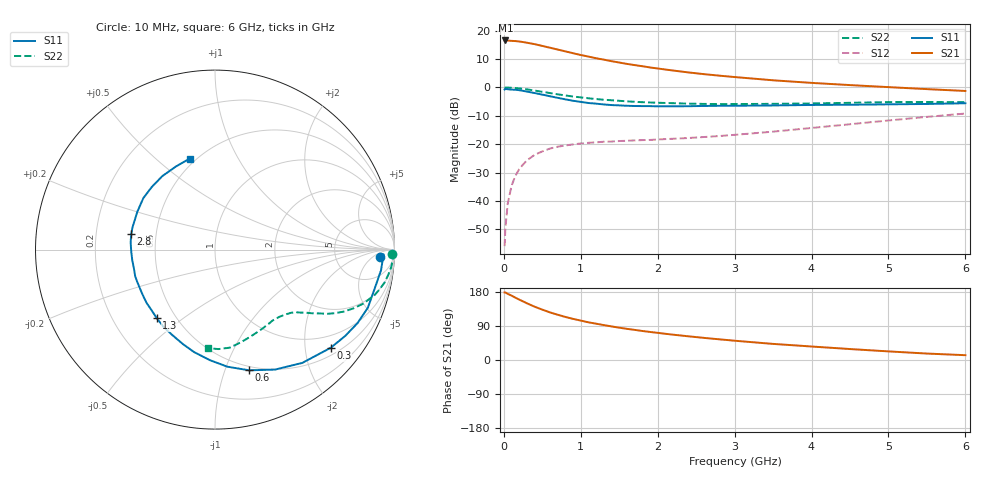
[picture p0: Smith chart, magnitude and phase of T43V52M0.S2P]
! Infineon Technologies  Discrete & RF Semiconductors
! BFR182T
! Si NPN RF Bipolar Junction Transistor in SC75
! VCE = 3.5 V  IC = 2 mA
! Common Emitter S-Parameters:  October  1999
# GHz  S  MA  R  50
!  f  S11  S21  S12  S22
! GHz  MAG  ANG  MAG  ANG  MAG  ANG  MAG  ANG
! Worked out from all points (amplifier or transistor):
!   36 points, 10 MHz to 6 GHz, reference 50 ohm
!   highest |S21| = 16.5 dB at 20 MHz (marker M1)
!   |S21| within 3 dB of that: start of sweep to 668.4 MHz
!   unconditionally stable (mu >= 1): 1.998 GHz to 4.334 GHz
!   at 250 MHz: K = 0.14, MSG = 21.6 dB, |S12| = -27.2 dB
!   at 1.4 GHz: K = 0.77, MSG = 14.2 dB, |S12| = -19.1 dB
!   at 6 GHz: K = 0.82, MSG = 4.0 dB, |S12| = -9.2 dB
!   lowest NFmin = 1.10 dB at 450 MHz
!   S11 on the Smith chart (normalised r, x): 10 MHz: 19, -10; 300 MHz: 0.67, -2.57; 600 MHz: 0.46, -1.21; 1.3 GHz: 0.39, -0.40; 2.8 GHz: 0.36, +0.08; 6 GHz: 0.46, +0.65
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0.01  0.9206 -2.5  6.654 178.3  0.0016 85.7  0.9888 -1.3
0.02  0.9395 -1.6  6.722 178.2  0.0033 97.7  0.9905 -1.1
0.05  0.9321 -7.1  6.688 174.7  0.0089 88.3  0.9931 -2.9
0.1  0.9161 -13.5  6.611 169.9  0.0185 83.3  0.9864 -5.7
0.15  0.9112 -20.8  6.555 164.5  0.0278 78.2  0.9749 -8.4
0.2  0.8935 -27.3  6.449 159.4  0.0364 76.1  0.9623 -11.0
0.3  0.8456 -40.3  6.126 149.7  0.0519 68.4  0.9255 -15.8
0.4  0.7969 -52.4  5.787 140.7  0.065 62.4  0.881 -19.9
0.5  0.7476 -63.4  5.385 132.9  0.0747 57.1  0.8379 -23.0
0.6  0.699 -74.2  5.006 125.6  0.0839 53.1  0.7964 -25.7
0.8  0.6165 -92.7  4.319 113.6  0.095 47.0  0.7224 -29.7
0.9  0.5825 -101.6  4.004 108.5  0.0993 45.3  0.6912 -31.0
1.1  0.5318 -116.7  3.494 99.4  0.1058 42.3  0.6441 -33.4
1.3  0.5011 -130.5  3.089 92.1  0.1106 41.0  0.6071 -35.3
1.6  0.4752 -148.0  2.597 82.2  0.115 40.4  0.5688 -37.8
1.9  0.4686 -161.7  2.25 74.0  0.1189 42.0  0.5433 -41.0
2.2  0.4648 -172.9  1.986 66.8  0.1248 44.2  0.5278 -43.9
2.8  0.4746 169.7  1.614 54.6  0.1393 49.6  0.5089 -51.1
3.5  0.4816 153.8  1.336 42.5  0.1664 55.4  0.5144 -60.1
4.5  0.4957 135.3  1.1 28.9  0.2248 58.9  0.536 -74.2
5.5  0.5116 115.2  0.934 17.0  0.3032 57.0  0.5546 -88.0
6  0.5263 105.6  0.867 12.7  0.347 54.1  0.5499 -94.3
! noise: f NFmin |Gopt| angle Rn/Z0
0.45  1.1  0.42  29  0.36
0.9  1.2  0.4  58  0.3
1.8  1.85  0.32  126  0.22
